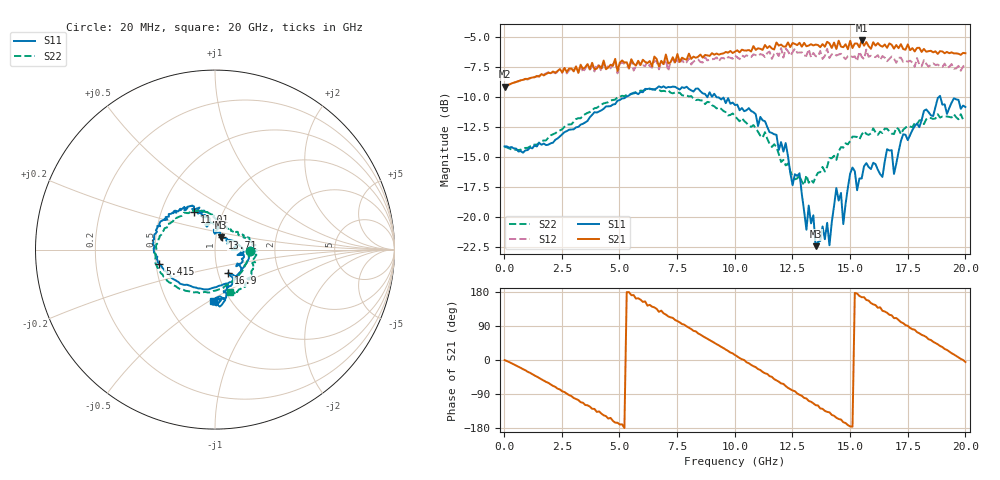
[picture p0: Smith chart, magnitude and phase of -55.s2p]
!Agilent Technologies,N5230A,US43500223,A.07.50.48
!Agilent N5230A: A.07.50.48
!Date: Tuesday, November 17, 2015 12:09:06
!Correction: S11(Full 2 Port(1,2))
!S21(Full 2 Port(1,2))
!S12(Full 2 Port(1,2))
!S22(Full 2 Port(1,2))
!S2P File: Measurements: S11, S21, S12, S22:
# Hz S  dB  R 50
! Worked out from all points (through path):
!   201 points, 20 MHz to 20 GHz, reference 50 ohm
!   highest |S21| = -5.32 dB at 15.5 GHz (marker M1); lowest = -9.2 dB at 20 MHz (marker M2)
!   group delay of S21, straight-line fit = 101 ps
!   lowest |S11| = -22.5 dB at 13.51 GHz (marker M3), VSWR 1.16, Z = 52.9 + j7.23 ohm
!   |S11| at or under -10 dB: start of sweep to 5.308 GHz; 9.192 GHz to 18.87 GHz (9.675 GHz wide, 69 % of centre); 18.91 GHz to end of sweep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
!   |S22| runs from -17.4 to -9.4 dB; largest |S21 - S12| = 0.12
!   S11 on the Smith chart (normalised r, x): 20 MHz: 1.49, -0.02; 5.415 GHz: 0.52, -0.09; 11.01 GHz: 0.73, +0.32; 13.71 GHz: 1.08, +0.15; 16.9 GHz: 1.11, -0.30; 20 GHz: 0.84, -0.52
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2e7  -14.14 -1.7  -9.18 -0.2  -9.19 -0.3  -14.19 -1.5
1.9181e9  -14.00 -77.0  -8.01 -60.4  -7.96 -62.0  -13.40 -75.9
3.4166e9  -12.26 -123.7  -7.69 -112.8  -7.98 -117.2  -11.59 -115.2
5.4146e9  -9.91 -165.5  -7.62 179.0  -7.68 175.7  -9.80 -152.8
6.7133e9  -9.14 174.7  -7.49 127.0  -7.73 124.1  -9.44 -170.9
8.012e9  -9.36 157.7  -6.42 85.3  -6.80 80.4  -9.99 167.7
1.001e10  -10.70 131.2  -6.25 13.1  -6.58 7.2  -11.63 128.5
1.1009e10  -12.45 119.2  -5.97 -24.0  -6.62 -29.9  -12.93 108.3
1.23077e10  -14.97 99.9  -5.48 -73.5  -6.22 -79.2  -15.57 79.3
1.28072e10  -16.38 96.9  -5.51 -91.8  -6.33 -96.4  -16.60 65.2
1.31069e10  -21.09 90.5  -5.81 -101.6  -6.61 -108.7  -16.55 52.6
1.34066e10  -19.89 73.7  -5.74 -114.3  -6.37 -121.1  -17.17 49.2
1.35065e10  -22.45 64.5  -5.67 -119.2  -6.63 -125.4  -16.70 40.9
1.37063e10  -22.02 58.7  -5.88 -127.7  -6.20 -133.7  -16.29 40.2
1.41059e10  -22.38 25.3  -5.57 -138.1  -6.78 -149.0  -15.11 28.7
1.44056e10  -17.61 19.0  -6.04 -152.4  -6.58 -160.1  -15.26 23.2
1.47053e10  -20.61 -0.7  -5.88 -164.2  -6.69 -171.3  -14.25 20.6
1.55045e10  -16.81 -6.2  -5.32 165.8  -6.69 158.5  -13.16 6.3
1.67033e10  -14.48 -49.7  -5.57 119.4  -6.86 114.7  -12.89 -10.5
1.69031e10  -16.44 -61.3  -6.01 110.4  -6.83 102.0  -13.12 -13.6
1.82018e10  -11.18 -77.1  -6.03 64.1  -6.96 58.3  -12.29 -41.9
2e10  -10.86 -91.7  -6.39 -5.2  -7.35 -14.1  -11.93 -70.3
